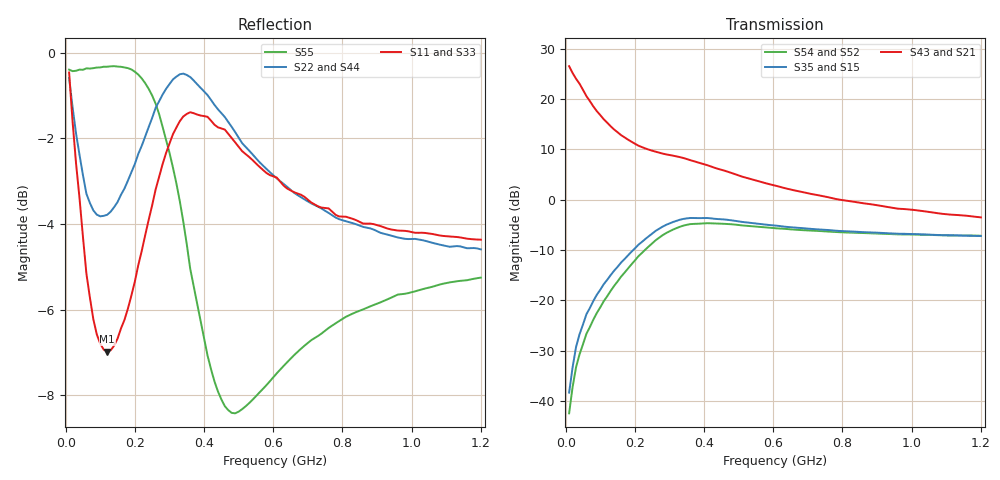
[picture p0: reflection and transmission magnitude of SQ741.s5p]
!  POLYFET RF DEVICES
!  SQ741 (EACH SIDE)
!  S PARAMETERS
!  VDS=50V, IDQ=200mA
!AWR Design Environment (2053) Wed Feb 04 15:38:52 2004
!freq-unit  param-type  data-format  keyword  impedance-ohms
# MHz  S  MA  R  50
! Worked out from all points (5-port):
!   120 points, 10 MHz to 1.2 GHz, reference 50 ohm
!   strongest paths, dB at 10 MHz, 310 MHz, 610 MHz, 910 MHz, 1.2 GHz:
!     S43: 26.5, 8.7, 2.7, -1.2, -3.5
!     S21: 26.5, 8.7, 2.7, -1.2, -3.5
!     S35: -38.3, -4.5, -5.2, -6.6, -7.2
!     S15: -38.3, -4.5, -5.2, -6.6, -7.2
!     S54: -42.5, -6.0, -5.7, -6.8, -7.2
!     S52: -42.5, -6.0, -5.7, -6.8, -7.2
!   lowest |S11| = -7.0 dB at 120 MHz (marker M1), VSWR 2.62, Z = 50.4 - j50.3 ohm
!   |S11| at or under -10 dB: nowhere
